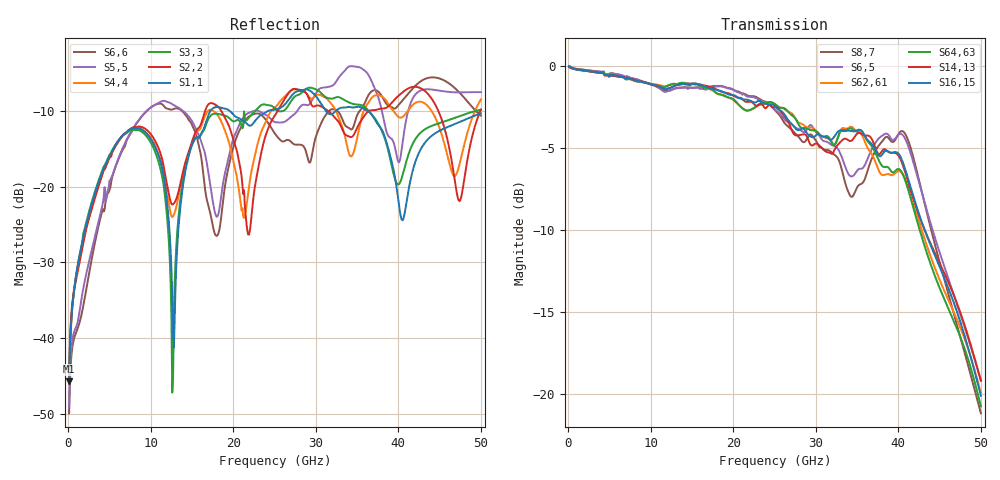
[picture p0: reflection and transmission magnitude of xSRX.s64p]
! DAC39RF10ACK
! 256-pin FCBGA package
! Texas Instruments 8/20/2022
! Port[1]  = 0SRXN_BGA
! Port[2]  = 0SRXN_DIE
! Port[3]  = 0SRXP_BGA
! Port[4]  = 0SRXP_DIE
! Port[5]  = 1SRXN_BGA
! Port[6]  = 1SRXN_DIE
! Port[7]  = 1SRXP_BGA
! Port[8]  = 1SRXP_DIE
! Port[9]  = 2SRXN_BGA
! Port[10]  = 2SRXN_DIE
! Port[11]  = 2SRXP_BGA
! Port[12]  = 2SRXP_DIE
! Port[13]  = 3SRXN_BGA
! Port[14]  = 3SRXN_DIE
! Port[15]  = 3SRXP_BGA
! Port[16]  = 3SRXP_DIE
! Port[17]  = 4SRXN_BGA
! Port[18]  = 4SRXN_DIE
! Port[19]  = 4SRXP_BGA
! Port[20]  = 4SRXP_DIE
! Port[21]  = 5SRXN_BGA
! Port[22]  = 5SRXN_DIE
! Port[23]  = 5SRXP_BGA
! Port[24]  = 5SRXP_DIE
! Port[25]  = 6SRXN_BGA
! Port[26]  = 6SRXN_DIE
! Port[27]  = 6SRXP_BGA
! Port[28]  = 6SRXP_DIE
! Port[29]  = 7SRXN_BGA
! Port[30]  = 7SRXN_DIE
! Port[31]  = 7SRXP_BGA
! Port[32]  = 7SRXP_DIE
! Port[33]  = 8SRXN_BGA
! Port[34]  = 8SRXN_DIE
! Port[35]  = 8SRXP_BGA
! Port[36]  = 8SRXP_DIE
! Port[37]  = 9SRXN_BGA
! Port[38]  = 9SRXN_DIE
! Port[39]  = 9SRXP_BGA
! Port[40]  = 9SRXP_DIE
! Port[41]  = 10SRXN_BGA
! Port[42]  = 10SRXN_DIE
! Port[43]  = 10SRXP_BGA
! Port[44]  = 10SRXP_DIE
! Port[45]  = 11SRXN_BGA
! Port[46]  = 11SRXN_DIE
! Port[47]  = 11SRXP_BGA
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# Hz	S	MA	R	50.000000
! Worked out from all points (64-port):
!   500 points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, 100 MHz to 50 GHz, reference 50 ohm
!   strongest paths, dB at 100 MHz, 12.6 GHz, 25.1 GHz, 37.6 GHz, 50 GHz:
!     S16,15: 0.0, -1.3, -2.5, -5.5, -20.1
!     S14,13: -0.1, -1.3, -2.5, -5.4, -19.2
!     S64,63: 0.0, -1.1, -2.4, -5.7, -20.7
!     S62,61: 0.0, -1.1, -2.4, -6.4, -19.9
!     S6,5: 0.0, -1.5, -2.7, -4.5, -19.2
!     S8,7: 0.0, -1.5, -2.8, -4.9, -21.2
!   lowest |S11| = -45.6 dB at 100 MHz (marker M1), VSWR 1.01, Z = 50.4 + j0.297 ohm
!   |S11| at or under -10 dB: start of sweep to 17.25 GHz; 19.54 GHz to 24.27 GHz (4.727 GHz wide, 21.6 % of centre); 36.21 GHz to end of sweep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
